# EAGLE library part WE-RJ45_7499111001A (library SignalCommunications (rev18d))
Order Code 7499111001A Design THT xBase-T 10/100/1000 Base-T Ports 1x1 Application Standard Tab Position UP LED (Left-Right) NONE EMI Fingers Yes Details see: http://katalog.we-online.de/en/pbs/WE-LAN_RJ45/7499111000A? Created by Yingchun Shan 2016-08-29 2016 (C) Würth Elektronik
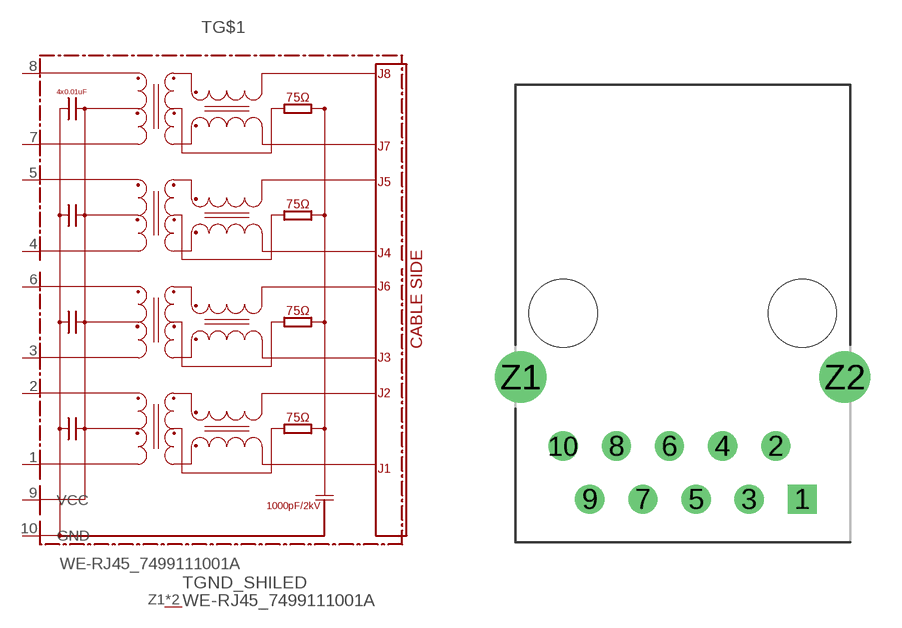
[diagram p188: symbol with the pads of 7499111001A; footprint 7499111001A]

Designator prefix T; gates G$1=7499111001A GND_SHILED=GND_PIN

## WE-RJ45_7499111001A  [7499111001A]
1  G$1:1
2  G$1:2
3  G$1:3
4  G$1:4
5  G$1:5
6  G$1:6
7  G$1:7
8  G$1:8
9  G$1:VCC
10  G$1:GND
Z1  GND_SHILED:1  pwr
Z2  GND_SHILED:1  pwr

## Footprint 7499111001A (pad centres in mm)
drill 0.89 square: 1 5.715,-8.89
drill 0.89: 2 4.445,-6.35; 3 3.175,-8.89; 4 1.905,-6.35; 5 0.635,-8.89; 6 -0.635,-6.35; 7 -1.905,-8.89; 8 -3.175,-6.35; 9 -4.445,-8.89; 10 -5.715,-6.35
drill 1.63: Z1 -7.745,-3.05; Z2 7.745,-3.05
hole 3.25 at -5.715,0
hole 3.25 at 5.715,0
